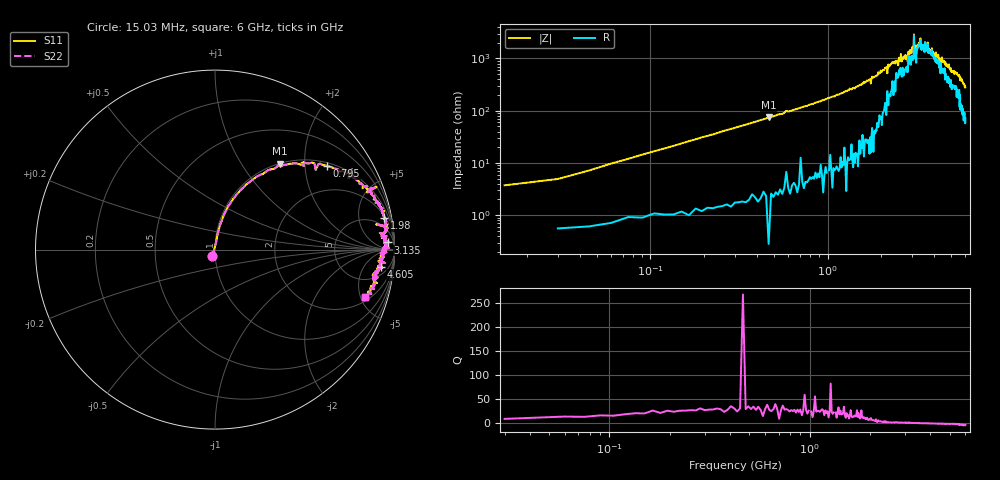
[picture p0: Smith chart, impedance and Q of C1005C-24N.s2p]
!	Network	Analyzer	HP8753E.07.74:	Oct	30	2002	Serial	No.	JP38451487
!	Hewlett-Packard
!	7	Sep	2009	9:00:17
!	Frequency	S11	S21	S12	S22
#	HZ	S	RI	R	50
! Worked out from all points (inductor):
!   400 points, 15.03 MHz to 6 GHz, reference 50 ohm
!   read as one part in series: L = 25.4 nH near 45.03 MHz
!   highest Q = 30.9 at 465 MHz (marker M1), where L = 25.8 nH
!   self-resonance near 3.451 GHz
!   S11 on the Smith chart (normalised r, x): 15.03 MHz: 0.97, -0.07; 795 MHz: 1.11, +2.61; 1.98 GHz: 2, +10; 3.135 GHz: 24, +27; 4.605 GHz: 9, -13; 6 GHz: 2.44, -5.42
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1.502992e7  -0.0141 -0.0358  1.01 0.0358  1.01 0.0358  -0.0141 -0.0358
1.650292e8  0.0719 0.24  0.928 -0.24  0.928 -0.24  0.0719 0.24
4.650277e8  0.363 0.479  0.637 -0.479  0.637 -0.479  0.363 0.479
7.95026e8  0.625 0.464  0.375 -0.464  0.375 -0.464  0.625 0.464
1.020025e9  0.746 0.415  0.254 -0.415  0.254 -0.415  0.746 0.415
1.98002e9  0.943 0.174  0.0567 -0.174  0.0567 -0.174  0.943 0.174
2.01002e9  0.947 0.166  0.0531 -0.166  0.0531 -0.166  0.947 0.166
2.595017e9  0.954 0.0634  0.0458 -0.0634  0.0458 -0.0634  0.954 0.0634
2.835016e9  0.927 0.0766  0.0727 -0.0766  0.0727 -0.0766  0.927 0.0766
3.015015e9  0.966 0.0462  0.0343 -0.0462  0.0343 -0.0462  0.966 0.0462
3.045015e9  0.944 0.0468  0.0556 -0.0468  0.0556 -0.0468  0.944 0.0468
3.075015e9  0.968 0.00888  0.0324 -0.00888  0.0324 -0.00888  0.968 0.00888
3.090015e9  0.951 0.0353  0.0486 -0.0353  0.0486 -0.0353  0.951 0.0353
3.135014e9  0.963 0.0398  0.0372 -0.0398  0.0372 -0.0398  0.963 0.0398
3.165014e9  0.943 0.0537  0.0572 -0.0537  0.0572 -0.0537  0.943 0.0537
3.345013e9  0.963 0.0133  0.0373 -0.0133  0.0373 -0.0133  0.963 0.0133
3.405013e9  0.937 0.00702  0.0631 -0.00702  0.0631 -0.00702  0.937 0.00702
3.675012e9  0.955 -0.0146  0.045 0.0146  0.045 0.0146  0.955 -0.0146
4.00501e9  0.938 -0.0446  0.0616 0.0446  0.0616 0.0446  0.938 -0.0446
4.605007e9  0.927 -0.0972  0.0731 0.0972  0.0731 0.0972  0.927 -0.0972
5.010005e9  0.902 -0.122  0.0976 0.122  0.0976 0.122  0.902 -0.122
6e9  0.833 -0.263  0.167 0.263  0.167 0.263  0.833 -0.263
